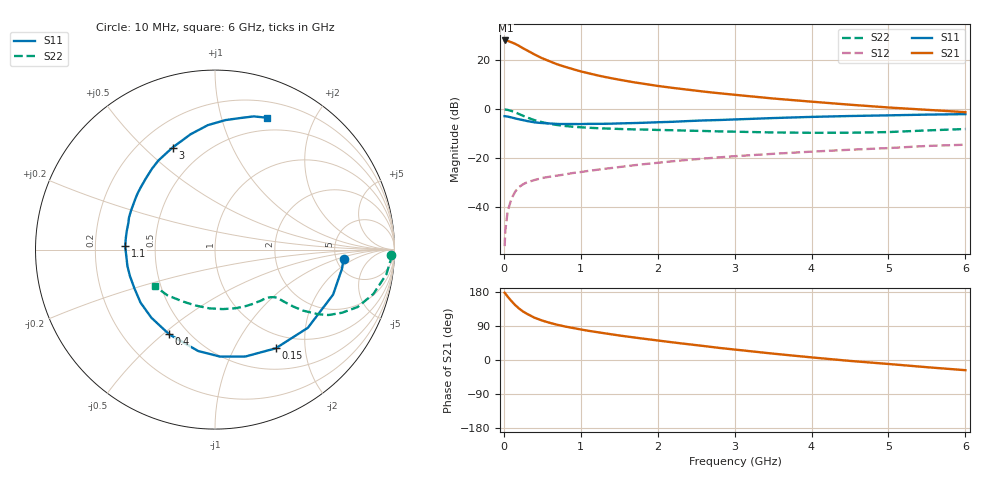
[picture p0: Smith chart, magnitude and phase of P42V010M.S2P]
! SIEMENS Small Signal Semiconductors
! BFP182
! Si NPN RF Bipolar Junction Transistor in SOT143
! VCE = 2 V  IC = 10 mA
! Common Emitter S-Parameters:  March  1996
# GHz  S  MA  R  50
!  f  S11  S21  S12  S22
! GHz  MAG  ANG  MAG  ANG  MAG  ANG  MAG  ANG
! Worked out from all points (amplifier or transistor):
!   36 points, 10 MHz to 6 GHz, reference 50 ohm
!   highest |S21| = 28.0 dB at 20 MHz (marker M1)
!   |S21| within 3 dB of that: start of sweep to 239.5 MHz
!   unconditionally stable (mu >= 1): 1.12 GHz to 5.373 GHz
!   at 250 MHz: K = 0.33, MSG = 27.7 dB, |S12| = -30.7 dB
!   at 1.4 GHz: K = 1.10, MAG = 16.4 dB, |S12| = -24.0 dB
!   at 6 GHz: K = 0.94, MSG = 6.6 dB, |S12| = -14.5 dB
!   lowest NFmin = 1.50 dB at 450 MHz
!   S11 on the Smith chart (normalised r, x): 10 MHz: 5.81, -1.26; 150 MHz: 0.79, -1.49; 400 MHz: 0.40, -0.52; 1.1 GHz: 0.33, +0.02; 3 GHz: 0.34, +0.61; 6 GHz: 0.36, +1.41
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0.01  0.718 -4.2  24.9 177.5  0.0016 84.8  0.9805 -1.6
0.02  0.7157 -8.5  25.18 175.2  0.0034 82.0  0.981 -3.3
0.05  0.7041 -20.9  24.67 167.1  0.0083 83.3  0.9647 -8.2
0.1  0.6763 -40.1  23.04 155.3  0.015 70.0  0.9167 -15.6
0.15  0.6457 -58.4  21.37 144.4  0.021 62.8  0.8569 -21.9
0.2  0.6193 -74.1  19.41 135.5  0.0259 58.8  0.7909 -26.4
0.25  0.5968 -87.3  17.42 128.0  0.0293 54.5  0.7309 -29.9
0.3  0.5728 -99.4  15.84 121.9  0.0321 50.8  0.6775 -32.1
0.4  0.5366 -118.4  13.02 111.5  0.0358 47.1  0.5947 -34.8
0.5  0.5194 -133.0  10.89 104.0  0.0394 44.4  0.5403 -36.0
0.6  0.5092 -144.6  9.412 97.9  0.0419 43.6  0.5012 -36.7
0.7  0.4982 -154.3  8.144 92.7  0.0442 43.8  0.4723 -37.2
0.9  0.4965 -169.4  6.526 84.4  0.0498 43.8  0.4371 -37.9
1.1  0.5006 177.9  5.397 77.0  0.055 44.2  0.4176 -39.4
1.3  0.5023 168.1  4.576 70.8  0.0604 44.4  0.4037 -41.2
1.6  0.5158 155.1  3.741 62.0  0.0687 44.8  0.3894 -44.8
2.2  0.5521 134.5  2.707 46.4  0.0865 43.2  0.371 -54.1
3  0.6158 112.6  1.962 27.6  0.1095 38.4  0.3466 -70.4
3.5  0.6571 101.9  1.648 16.8  0.1225 34.7  0.3344 -82.4
4.5  0.7239 85.4  1.231 -2.4  0.1484 27.3  0.33 -109.4
5.5  0.7729 73.8  0.968 -19.0  0.1772 20.0  0.3678 -136.2
6  0.7904 68.3  0.867 -26.9  0.188 15.2  0.393 -148.9
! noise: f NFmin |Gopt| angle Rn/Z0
0.45  1.5  0.26  43  0.28
0.9  1.6  0.24  87  0.22
1.8  2.1  0.2  170  0.2
